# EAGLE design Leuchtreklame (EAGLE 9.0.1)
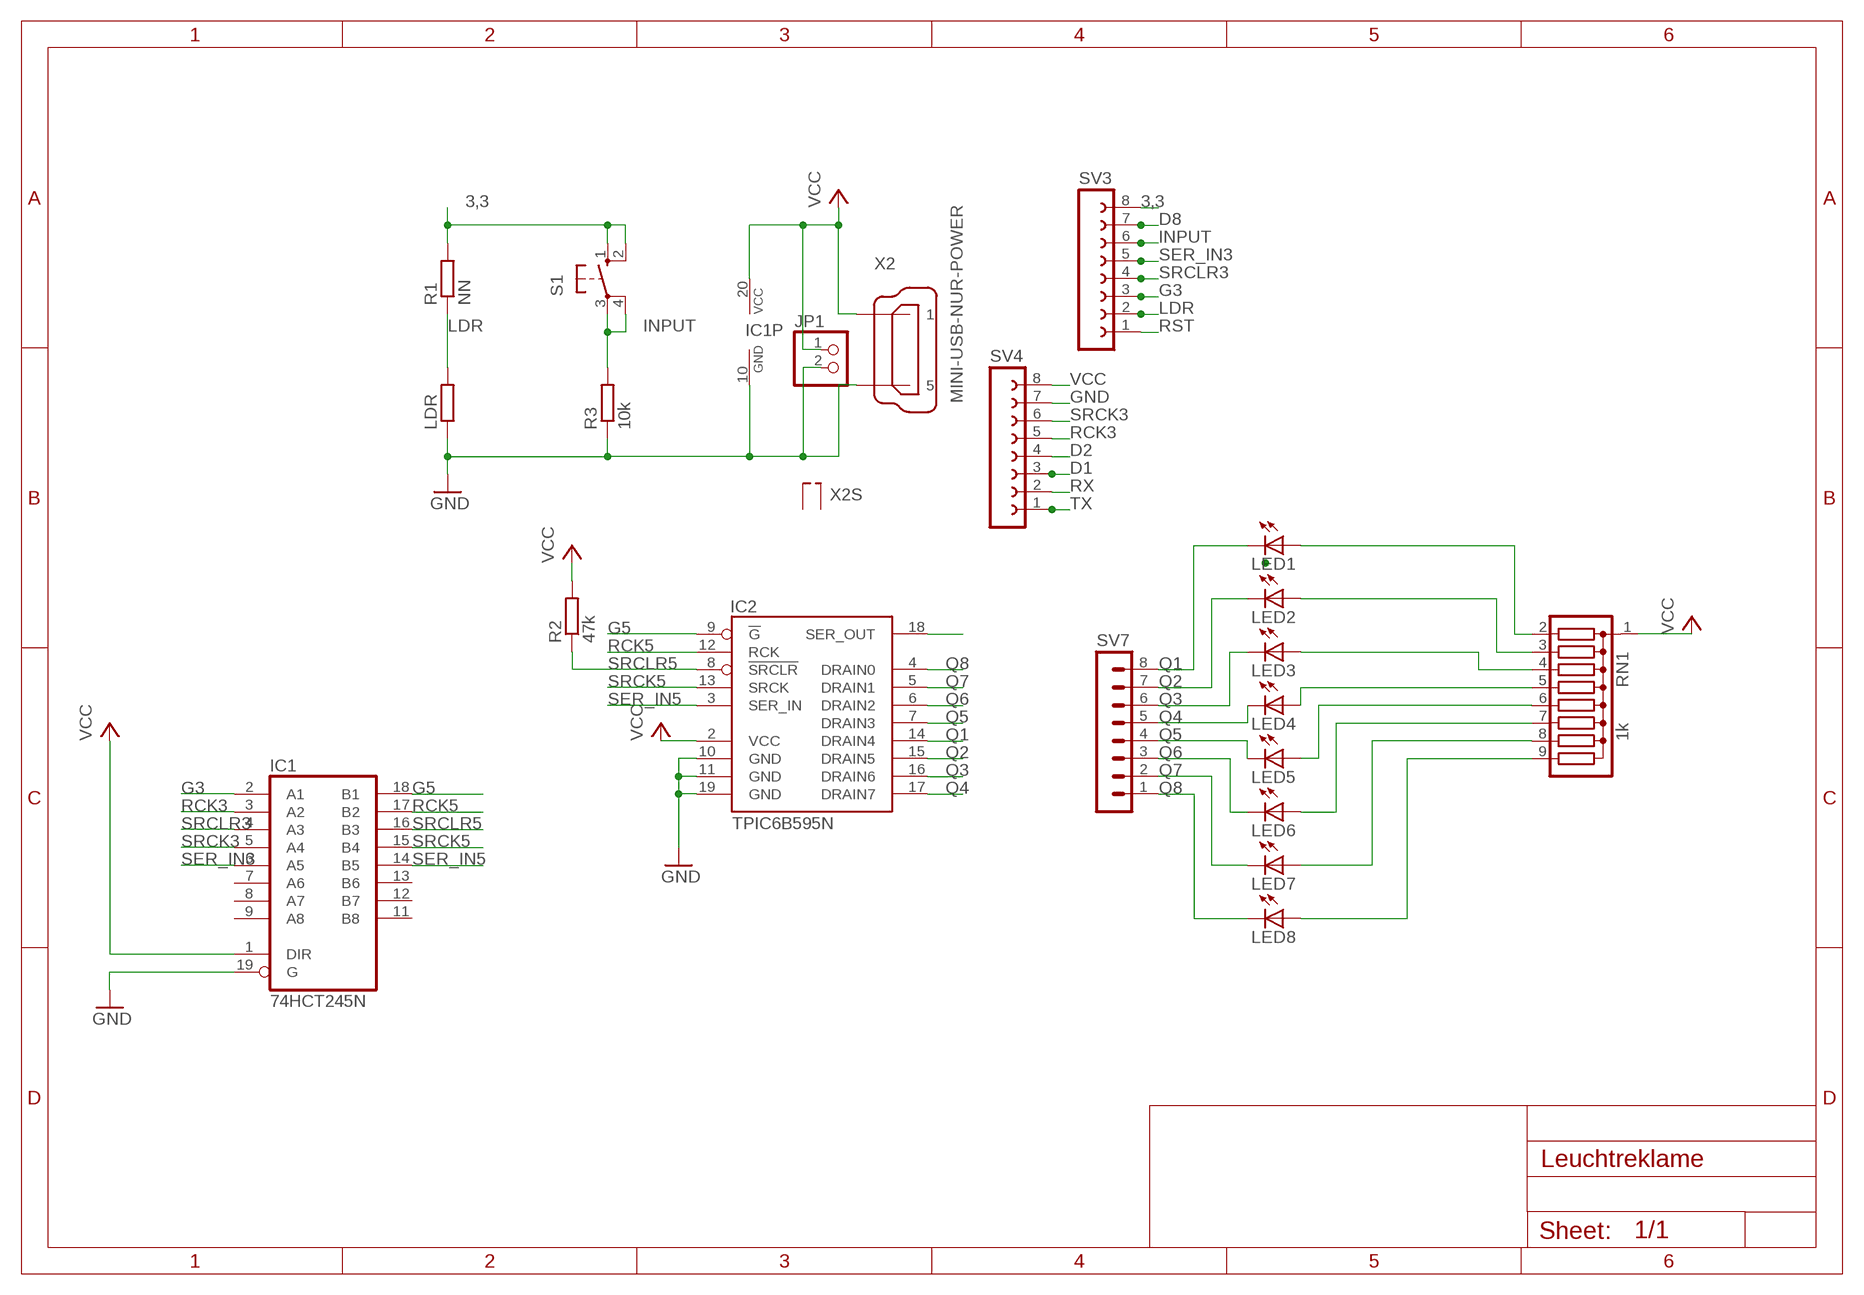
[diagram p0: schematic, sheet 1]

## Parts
IC1  74HCT245N  [DIL20]
IC2  TPIC6B595N  [DIL20]
JP1  PINHD-1X2  [1X02]
LDR  R-EU_0204/5  [0204/5]
LED1  LED3MM  [LED3MM]
LED2  LED3MM  [LED3MM]
LED3  LED3MM  [LED3MM]
LED4  LED3MM  [LED3MM]
LED5  LED3MM  [LED3MM]
LED6  LED3MM  [LED3MM]
LED7  LED3MM  [LED3MM]
LED8  LED3MM  [LED3MM]
R1  NN  R-EU_0207/10  [0207/10]
R2  47k  R-EU_0207/10  [0207/10]
R3  10k  R-EU_0207/10  [0207/10]
RN1  1k  G08R  [SIL9]
S1  10-XX  [B3F-10XX]
SV3  FE08-1  [FE08]
SV4  FE08-1  [FE08]
SV7  MA08-1  [MA08-1]
X2  MINI-USB-NUR-POWER  [MINI-USB-POWER]

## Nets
3,3: R1.2 S1.1(S) S1.2(S1) SV3.8
D1: SV4.3
D2: SV4.4
D8: SV3.7
G3: IC1.2(A1) SV3.3
G5: IC1.18(B1) IC2.9(!G)
GND: IC1.10(GND) IC1.19(G) IC2.10(GND) IC2.11(GND) IC2.19(GND) JP1.2 LDR.1 R3.1 SV4.7 X2.5
INPUT: R3.2 S1.3(P) S1.4(P1) SV3.6
LDR: LDR.2 R1.1 SV3.2
N$1: LED1.A RN1.2
N$2: LED2.A RN1.3
N$3: LED3.A RN1.4
N$4: LED4.A RN1.5
N$9: LED5.A RN1.6
N$11: LED6.A RN1.7
N$12: LED7.A RN1.8
N$13: IC2.18(SER_OUT)
N$14: LED8.A RN1.9
Q1: IC2.14(DRAIN4) LED1.K(C) SV7.8
Q2: IC2.15(DRAIN5) LED2.K(C) SV7.7
Q3: IC2.16(DRAIN6) LED3.K(C) SV7.6
Q4: IC2.17(DRAIN7) LED4.K(C) SV7.5
Q5: IC2.7(DRAIN3) LED5.K(C) SV7.4
Q6: IC2.6(DRAIN2) LED6.K(C) SV7.3
Q7: IC2.5(DRAIN1) LED7.K(C) SV7.2
Q8: IC2.4(DRAIN0) LED8.K(C) SV7.1
RCK3: IC1.3(A2) SV4.5
RCK5: IC1.17(B2) IC2.12(RCK)
RST: SV3.1
RX: SV4.2
SER_IN3: IC1.6(A5) SV3.5
SER_IN5: IC1.14(B5) IC2.3(SER_IN)
SRCK3: IC1.5(A4) SV4.6
SRCK5: IC1.15(B4) IC2.13(SRCK)
SRCLR3: IC1.4(A3) SV3.4
SRCLR5: IC1.16(B3) IC2.8(!SRCLR) R2.1
TX: SV4.1
VCC: IC1.1(DIR) IC1.20(VCC) IC2.2(VCC) JP1.1 R2.2 RN1.1 SV4.8 X2.1
Unconnected: IC1.7(A6) IC1.8(A7) IC1.9(A8) IC1.11(B8) IC1.12(B7) IC1.13(B6) X2.M1(S1) X2.M2(S2)

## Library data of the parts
IC1 = 74xx-eu:74*245: Octal BUS TRANSCEIVER, 3-state
IC2 = TPIC6B595:TPIC6B595
JP1 = 1a BK_Hennef:PINHD-1X2: PIN HEADER
LDR R1-R3 = 1a BK_Hennef:R-EU_: RESISTOR, European symbol
LED1-LED8 = 1a BK_Hennef:LED: LED
RN1 = resistor-sil:G08R: SIL RESISTOR; OC_FARNELL: unknown; OC_NEWARK: unknown
S1 = switch-omron:10-XX: OMRON SWITCH; MPN: B3F-1000; OC_FARNELL: 176432; OC_NEWARK: 36M3542
SV3 SV4 = con-lsta:FE08-1: FEMALE HEADER; OC_FARNELL: unknown; OC_NEWARK: unknown
SV7 = con-lstb:MA08-1: PIN HEADER; OC_FARNELL: unknown; OC_NEWARK: unknown
X2 = 1a BK_Hennef:MINI-USB-NUR-POWER: MINI USB-B R/A DIP 5pol. Reichelt Nr.: USB BWM

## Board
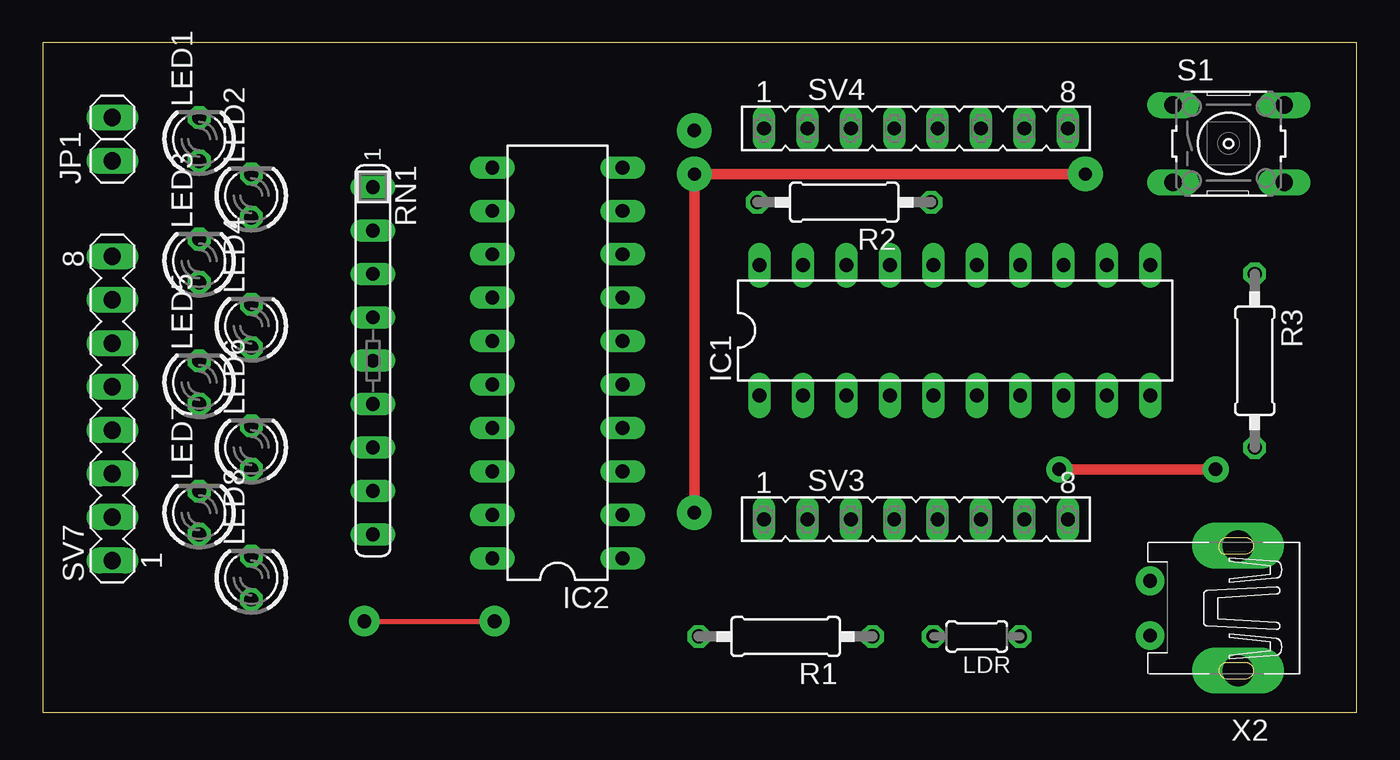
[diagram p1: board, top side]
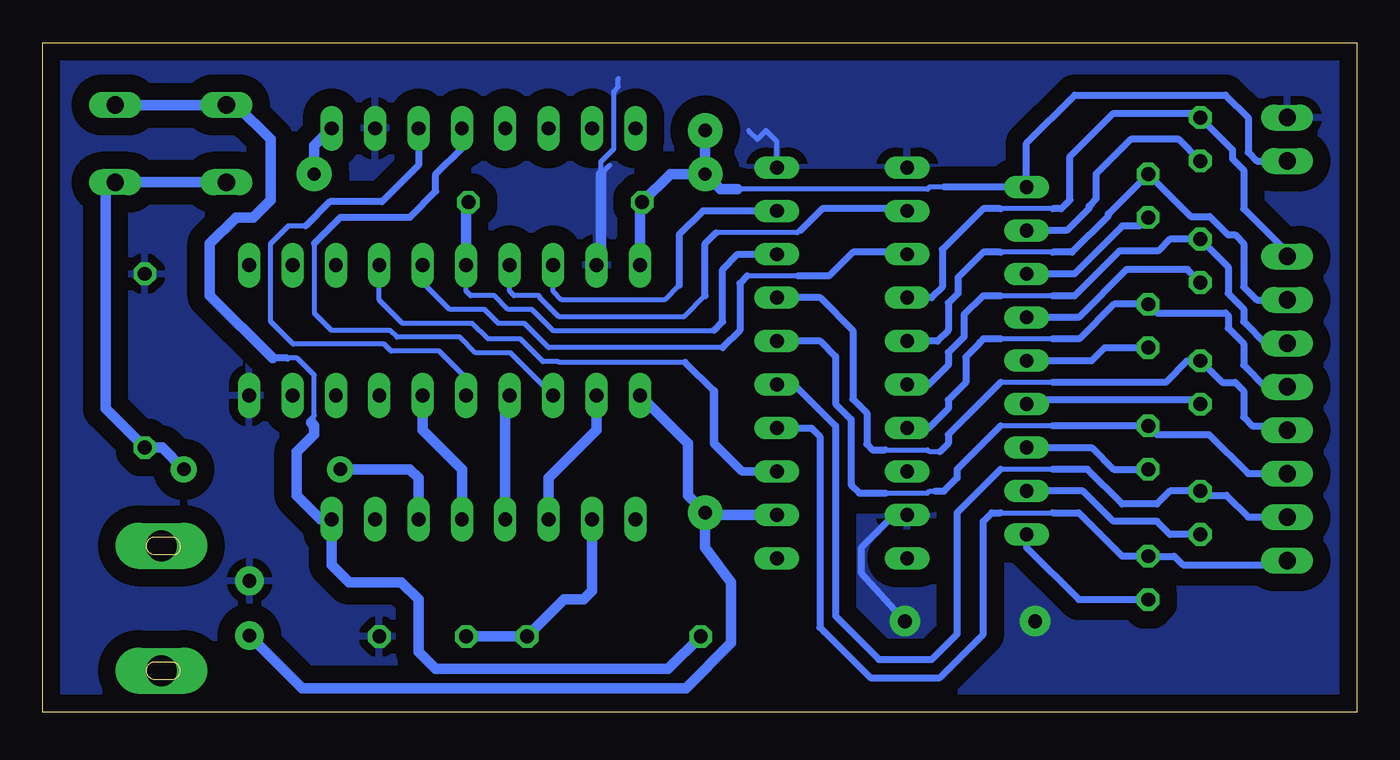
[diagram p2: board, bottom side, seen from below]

Size 76.83 x 39.17 mm. Coordinates in mm from the lower left corner, seen from the top.
Outline: 0,0 76.83,0 76.83,39.17 0,39.17 0,0
Copper layers (1*16): Top 0.035mm / dielectric 1.5mm / Bottom 0.035mm
Design rules "Bilex DRU *": minimum track width 12mil, minimum drill 30mil, track to track 20mil, track to pad 18mil, pad to pad 18mil, via to via 20mil, smd to smd 15mil, copper to edge 20mil, drill to drill 20mil, minimum pad ring 10mil, minimum via ring 8mil, stop-mask expansion 4mil, vias tented up to drill 0mil, thermal gap 20mil

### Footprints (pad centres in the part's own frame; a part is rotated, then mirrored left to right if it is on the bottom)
DIL20 = drill 0.813 long: 1 -11.43,-3.81; 2 -8.89,-3.81; 3 -6.35,-3.81; 4 -3.81,-3.81; 5 -1.27,-3.81; 6 1.27,-3.81; 7 3.81,-3.81; 8 6.35,-3.81; 9 8.89,-3.81; 10 11.43,-3.81; 11 11.43,3.81; 12 8.89,3.81; 13 6.35,3.81; 14 3.81,3.81; 15 1.27,3.81; 16 -1.27,3.81; 17 -3.81,3.81; 18 -6.35,3.81; 19 -8.89,3.81; 20 -11.43,3.81
1X02 = drill 1.016 long: 1 -1.27,0; 2 1.27,0
0204/5 = drill 0.813 octagon: 1 -2.54,0; 2 2.54,0
LED3MM = drill 0.813 octagon: A -1.27,0; K 1.27,0
0207/10 = drill 0.813 octagon: 1 -5.08,0; 2 5.08,0
SIL9 = drill 0.813 long: 1 -10.16,0; 2 -7.62,0; 3 -5.08,0; 4 -2.54,0; 5 0,0; 6 2.54,0; 7 5.08,0; 8 7.62,0; 9 10.16,0
B3F-10XX = drill 1.016 long: 1 -3.251,2.261; 2 3.251,2.261; 3 -3.251,-2.261; 4 3.251,-2.261
FE08 = drill 0.813 long: 1 -8.89,0; 2 -6.35,0; 3 -3.81,0; 4 -1.27,0; 5 1.27,0; 6 3.81,0; 7 6.35,0; 8 8.89,0
MA08-1 = drill 1.016 long: 1 -8.89,0; 2 -6.35,0; 3 -3.81,0; 4 -1.27,0; 5 1.27,0; 6 3.81,0; 7 6.35,0; 8 8.89,0
MINI-USB-POWER = drill 0.8 pad 1.676: 1 2.825,1.6; 5 2.825,-1.6 | drill 1.8 pad 2.2 long: M1 -2.325,3.65; M2 -2.325,-3.65

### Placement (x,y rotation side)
IC1  53.34,22.35 0 top
IC2  30.1,20.45 90 top
JP1  4.06,33.53 90 top
LDR  54.61,4.45 180 top
LED1  9.14,33.53 90 top
LED2  12.19,30.23 90 top
LED3  9.14,26.42 90 top
LED4  12.19,22.61 90 top
LED5  9.14,19.3 90 top
LED6  12.19,15.49 90 top
LED7  9.14,11.68 90 top
LED8  12.19,7.87 90 top
R1  43.43,4.45 180 top
R2  46.86,29.84 180 top
R3  70.87,20.57 270 top
RN1  19.3,20.57 270 top
S1  69.34,33.27 0 top
SV3  51.05,11.3 0 top
SV4  51.05,34.16 0 top
SV7  4.06,17.78 90 top
X2  67.56,6.1 180 top

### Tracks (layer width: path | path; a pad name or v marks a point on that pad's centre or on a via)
3,3
  Bottom 0.305: 61.15,16.95 61.15,17.17 60.96,17.36 60.96,19.73 61.96,20.73 62.52,20.73
  Bottom 0.406: 62.52,20.73 63.4,20.73
  Bottom 0.61: S1.2 S1.1 65.51,35.53 63.5,33.53 63.5,29.97 64.52,28.96 65.53,28.96 67.06,27.43 67.06,24.38 63.4,20.73 | R1.2 40.26,2.54 53.85,2.54 54.86,3.56 54.86,6.6 55.88,7.62 58.93,7.62 59.94,8.64 SV3.8 60.58,11.3 61.98,12.7 61.98,15.24 60.96,16.26 60.96,16.76 61.15,16.95
G3
  Bottom 0.61: SV3.3 47.24,13.72 44.45,16.51 IC1.2
G5
  Bottom 0.305: 39.62,24.99 40.49,24.13 46.48,24.13 46.99,24.64 IC1.18
  Bottom 0.406: IC2.9 38.23,29.34 39.62,27.94 39.62,24.99
GND  (via drill 0.8 pad 1.78)
  Top 0.305: v18.8,5.33 v26.42,5.33
  Bottom 0.305: IC2.10 33.91,33.4 34.54,34.04 35.05,33.53 35.56,34.04 | 43.69,32 44.2,31.5 | 44.2,26.42 IC1.19 | 44.2,28.96 44.2,32.22 43.43,32.98 43.43,36.32 43.18,36.58 43.18,37.08
  Bottom 0.406: v26.42,5.33 28.96,8.13 28.96,9.65 27.05,11.56 IC2.19
  Bottom 0.61: 44.2,31.5 44.2,28.96 44.2,26.42
  pour Bottom (isolate 1.016): 0,38.86 76.71,38.86 76.71,0 0,0
INPUT  (via drill 0.8 pad 1.52)
  Top 0.61: v59.44,14.22 v68.58,14.22
  Bottom 0.61: v68.58,14.22 69.85,15.49 R3.2 73.15,17.78 73.15,30.45 S1.4 S1.3 | SV3.6 54.86,13.72 55.37,14.22 v59.44,14.22
LDR
  Bottom 0.61: SV3.2 44.7,7.11 45.21,6.6 46.35,6.6 R1.1 LDR.2
N$1
  Bottom 0.406: LED1.A 10.41,33.53 13.21,33.53 15.24,31.5 15.24,30.03 15.65,29.62 15.65,29.51 16.96,28.19 RN1.2
N$2
  Bottom 0.406: LED2.A 12.7,28.45 13.72,28.45 16.51,25.65 RN1.3
N$3
  Bottom 0.406: LED3.A 9.91,25.91 13.46,25.91 16.26,23.11 RN1.4
N$4
  Bottom 0.406: RN1.5 15.49,20.57 14.73,21.34 LED4.A
N$9
  Bottom 0.406: LED5.A 9.4,18.29 19.05,18.29 RN1.6
N$11
  Bottom 0.406: RN1.7 15.49,15.49 14.22,14.22 LED6.A
N$12
  Bottom 0.406: LED7.A 10.92,10.41 11.68,11.18 14.22,11.18 16,12.95 RN1.8
N$14
  Bottom 0.406: RN1.9 19.3,9.65 16.26,6.6 LED8.A
Q1
  Bottom 0.305: 17.78,29.46 20.83,29.46
  Bottom 0.406: 20.83,29.46 21.84,29.46 24.23,27.08 24.23,24.89 24.87,24.26 IC2.14 | 17.78,29.46 17.27,29.46 16.76,29.97 16.76,32.51 14.22,35.05 9.4,35.05 LED1.K 9.02,34.67 7.26,32.92 7.26,32.39 6.6,31.73 6.6,29.46 4.06,26.92 SV7.8
Q2
  Bottom 0.305: 17.78,26.92 20.83,26.92
  Bottom 0.406: IC2.15 24.51,21.72 23.88,22.35 23.88,23.95 23.32,24.51 23.32,25.45 21.84,26.92 20.83,26.92 | 17.78,26.92 16.65,26.92 14.53,29.05 14.53,29.16 LED2.K 9.7,29.01 8.6,29.01 7.53,27.94 7.11,27.94 6.6,27.43 6.6,24.89 5.84,24.13 SV7.7
Q3
  Bottom 0.305: 20.83,24.38 17.78,24.38
  Bottom 0.406: IC2.16 25.02,19.18 23.88,20.32 23.88,21.06 22.96,21.97 22.96,23.27 21.84,24.38 20.83,24.38 | 17.78,24.38 16.49,24.38 13.87,27 11.61,27 10.92,27.69 LED3.K 7.52,26.06 7.52,24.51 6.6,23.6 6.6,22.86 5.33,21.59 SV7.6 4.32,21.84
Q4
  Bottom 0.305: 22.86,19.3 22.86,20.83 | 17.78,21.84 20.83,21.84
  Bottom 0.406: 17.78,21.84 16.23,21.84 14.2,23.88 LED4.K 11.68,23.37 7.67,23.37 7.64,23.34 7.52,23.22 7.52,22.48 6.6,21.57 6.6,20.32 5.33,19.05 SV7.5 | 20.83,21.84 21.84,21.84 22.05,21.64 22.05,21.59 22.86,20.78 22.86,19.3 23.88,18.29 23.88,17.78 25.02,16.64 IC2.17
Q5
  Bottom 0.305: 17.78,19.3 20.83,19.3 | 24.38,15.24 24.98,15.24 25.1,15.37 27.56,15.37
  Bottom 0.406: 17.78,19.3 11.18,19.3 9.91,20.57 LED5.K 7.87,19.3 7.11,19.3 6.6,18.8 6.6,17.27 6.1,16.76 4.32,16.76 SV7.4 | 20.83,19.3 23.88,16.26 23.88,15.75 24.38,15.24 | IC2.7 31.37,24.26 29.46,22.35 29.46,18.33 28.65,17.52 28.65,15.7 28.32,15.37 27.56,15.37
Q6
  Bottom 0.305: 17.78,16.76 20.83,16.76 | 24.64,12.95 24.98,12.95 25.1,12.83 27.55,12.83
  Bottom 0.406: 17.78,16.76 LED6.K 11.68,16.26 8.64,16.26 6.35,13.97 SV7.3 | 20.83,16.76 23.37,14.22 23.37,13.72 24.13,12.95 24.64,12.95 | IC2.6 31.37,21.72 30.48,20.83 30.48,18.06 29.57,17.14 29.57,13.31 29.08,12.83 27.55,12.83
Q7
  Bottom 0.305: 29.46,4.57 27.99,3.1 27.94,3.1 | 17.78,14.22 20.83,14.22
  Bottom 0.406: 17.78,14.22 15.75,14.22 13.72,12.19 11.68,12.19 10.92,12.95 LED7.K 8.89,12.7 7.62,12.7 6.35,11.43 SV7.2 | 20.83,14.22 23.37,11.68 23.37,4.57 24.84,3.1 27.94,3.1 30.48,5.64 30.48,16.76 32.89,19.18 IC2.5
Q8
  Bottom 0.305: 30.58,4.17 28.45,2.03 | 20.83,11.68 17.78,11.68
  Bottom 0.406: 17.78,11.68 16.26,11.68 13.72,9.14 LED8.K 10.67,9.14 10.16,8.64 4.32,8.64 SV7.1 | 20.83,11.68 21.34,11.68 21.84,11.18 21.84,4.57 24.38,2.03 28.45,2.03 31.39,4.98 31.39,16.15 31.88,16.64 IC2.4 | 31.13,4.71 30.58,4.17
RCK3
  Bottom 0.305: 52.32,33.02 SV4.5 | IC1.3 49.48,21.03 51.51,21.03 52.43,21.95 56.12,21.95 56.52,22.35 59.94,22.35 60.96,23.37 60.96,27.43
  Bottom 0.406: 52.32,33.02 53.85,31.5 53.85,30.48 55.37,28.96 59.44,28.96 60.96,27.43
RCK5
  Bottom 0.305: 32.51,28.19 32.6,28.19 32.72,28.07 37.47,28.07 | IC1.17 49.53,24.64 49.28,24.38 47.8,24.38 47.8,24.3 46.67,23.16 39.32,23.16 38.1,24.38
  Bottom 0.406: IC2.12 26.42,29.46 31.24,29.46 32.51,28.19 | 38.1,24.38 38.1,27.43 37.47,28.07
SER_IN3
  Bottom 0.61: SV3.5 52.32,14.22 54.61,16.51 IC1.6
SER_IN5
  Bottom 0.305: 39.27,20.47 46.64,20.47 46.69,20.52 47.58,20.52 48.9,21.84 50.8,21.84 51.71,22.76 55.78,22.76 57.15,24.13 IC1.14
  Bottom 0.406: 37.59,18.8 39.27,20.47
  Bottom 0.508: 37.59,18.8 37.59,15.75 35.94,14.1 IC2.3
SRCK3
  Bottom 0.305: 52.07,19.56 53.65,21.13 56.45,21.13 56.86,21.54 62.18,21.54 63.5,22.86 63.5,27.43 62.48,28.45 61.47,28.45
  Bottom 0.406: IC1.5 52.07,19.56 | SV4.6 54.86,32 57,29.87 60.05,29.87 61.47,28.45
SRCK5
  Bottom 0.305: IC1.15 54.36,25.91 54.36,24.89 53.03,23.57 51,23.57 50.19,22.76 48.67,22.76 47.24,21.34 37.08,21.34 | 32.65,25.53 35.64,25.53
  Bottom 0.406: IC2.13 26.42,26.92 29.46,26.92 30.86,25.53 32.65,25.53 | 35.64,25.53 36.07,25.1 36.07,22.35 37.08,21.34
SRCLR3
  Bottom 0.61: SV3.4 49.78,18.29 IC1.4
SRCLR5
  Bottom 0.305: 52.07,29.72 R2.1 | 37.59,22.35 47,22.35 48.22,23.57 49.61,23.57 50.42,24.38 51.82,24.38 52.07,24.64 IC1.16
  Bottom 0.406: 37.59,22.35 37.08,22.86 37.08,25.91 36.2,26.8 IC2.8
  Bottom 0.61: IC1.16 52.07,29.72
VCC  (via drill 0.76 pad 2.03, 0.8 pad 2.03)
  Top 0.61: v38.1,11.68 v38.1,31.5 v60.96,31.5
  Bottom 0.305: IC1.20 41.78,26.29 | v38.1,11.68 38.48,11.56 38.35,11.43 | 41.91,29.72 R2.2 | 24.13,30.73 24.98,30.73 25.1,30.61 36.2,30.61
  Bottom 0.406: 24.13,30.73 RN1.1 19.3,33.3 16.48,36.12 7.67,36.12 6.35,34.8 6.35,32.77 5.84,32.26 JP1.1
  Bottom 0.61: IC1.1 39.12,15.75 39.12,12.7 v38.1,11.68 38.1,9.65 36.58,7.62 36.58,4.06 39.22,1.42 61.66,1.42 X2.1 | IC2.2 38.48,11.56 | IC1.20 41.91,29.72 | 36.2,30.61 37.21,30.61 v38.1,31.5 | v38.1,31.5 40.13,31.5 R2.2 | SV4.8 60.96,33.15 v60.96,31.5 | v38.1,31.5 v38.1,34.04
